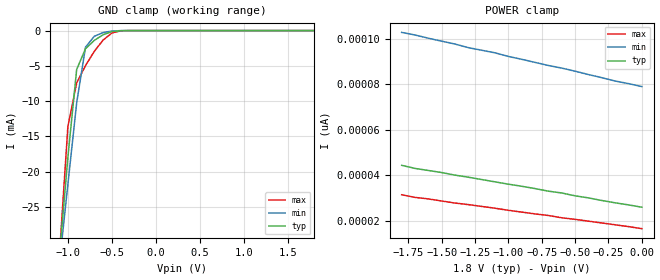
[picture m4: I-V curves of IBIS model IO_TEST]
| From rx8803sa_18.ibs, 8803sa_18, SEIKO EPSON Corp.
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[Model]   IO_TEST
Model_type Input
Enable Active-High
Polarity Non-Inverting
Vinh=1.44
Vinl=0.36
C_comp   5p   4p   6p
[Temperature Range] 25   85   -40
[Voltage Range]   1.8   1.6   2.0
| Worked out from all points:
|   GND clamp passes 1 mA (typ) near -0.65 V on its own axis
[GND Clamp]
-1.8V     -136.6mA   -117.3mA   -169.7mA
-1.1V     -32.43mA   -33.46mA   -32.61mA
-1V       -17.96mA   -21.79mA   -13.59mA
-900mV    -5.499mA   -10.22mA   -7.421mA
-800mV    -2.576mA   -2.362mA   -4.965mA
-700mV    -1.392mA   -807.3uA   -2.943mA
-600mV    -591.5uA   -281.9uA   -1.347mA
-500mV    -144.6uA   -61.93uA   -343.6uA
-400mV    -15.25uA   -7.313uA   -28.72uA
1.8V      25.81pA    81.4pA     14.78pA
[POWER Clamp]
-1.8V     44.34pA    102.8pA    31.38pA
-1.7V     42.97pA    101.6pA    30.24pA
-1.5V     41.15pA    98.91pA    28.65pA
-1.4V     40.02pA    97.66pA    27.74pA
-1.3V     39.11pA    96.07pA    27.06pA
-1.1V     37.06pA    93.79pA    25.47pA
-1V       36.04pA    92.2pA     24.56pA
-700mV    32.97pA    88.22pA    22.28pA
-600mV    32.17pA    87.08pA    21.26pA
-500mV    30.92pA    85.72pA    20.58pA
-200mV    27.85pA    81.4pA     18.19pA
0V        25.92pA    78.96pA    16.48pA
